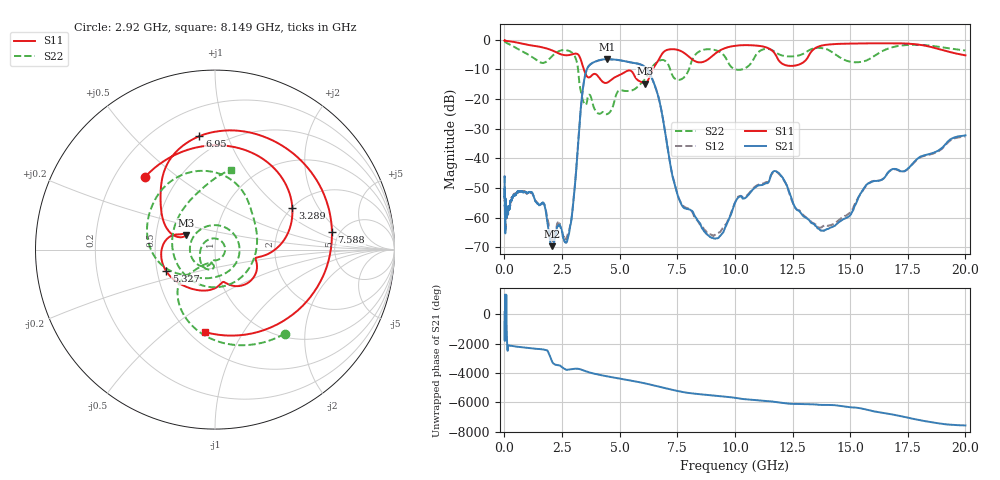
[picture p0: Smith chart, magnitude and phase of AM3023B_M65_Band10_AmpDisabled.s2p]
!Agilent Technologies,E8364B,MY43040894,A.07.50.67
!Agilent E8364B: A.07.50.67
!Date: Tuesday, October 27, 2020 10:50:51
!Correction: S11(Full 2 Port(1,2))
!S21(Full 2 Port(1,2))
!S12(Full 2 Port(1,2))
!S22(Full 2 Port(1,2))
!S2P File: Measurements: S11, S21, S12, S22:Log Frequency Sweep
# Hz S  dB  R 50
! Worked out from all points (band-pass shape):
!   3201 points, 10 MHz to 20 GHz, reference 50 ohm
!   highest |S21| = -6.60 dB at 4.447 GHz (marker M1); lowest = -69.6 dB at 2.06 GHz (marker M2)
!   |S21| within 3 dB of the highest: 3.602 GHz to 6.153 GHz (2.55 GHz wide, 52.3 % of centre)
!   lowest |S11| = -14.8 dB at 6.099 GHz (marker M3), VSWR 1.44, Z = 35.6 + j5.94 ohm
!   |S11| at or under -10 dB: 3.445 GHz to 6.435 GHz (2.99 GHz wide, 60.5 % of centre)
!   |S22| runs from -25.2 to -0.6 dB; largest |S21 - S12| = 0.0089
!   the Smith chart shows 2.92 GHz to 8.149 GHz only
!   S11 on the Smith chart (normalised r, x): 2.92 GHz: 0.33, +0.38; 3.289 GHz: 2.02, +1.22; 5.327 GHz: 0.56, -0.15; 6.95 GHz: 0.38, +0.80; 7.588 GHz: 4.33, +1.48; 8.149 GHz: 0.59, -0.70
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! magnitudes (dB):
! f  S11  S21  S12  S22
! 10 MHz  -0.3  -46.2  -45.8  -0.6
! 35.55 MHz  -0.3  -63.9  -63.7  -0.7
! 48.3 MHz  -0.3  -53.5  -57.0  -0.9
! 126.1 MHz  -0.5  -58.4  -58.4  -1.3
! 447.2 MHz  -0.8  -52.4  -52.2  -2.5
! 1.59 GHz  -2.5  -55.5  -55.4  -7.8
! 2.06 GHz  -3.6  -69.6  -67.6  -5.7
! 2.694 GHz  -5.3  -68.4  -66.7  -3.6
! 2.92 GHz  -5.0  -59.7  -60.0  -4.3
! 3.289 GHz  -6.2  -25.6  -25.6  -16.3
! 3.608 GHz  -12.6  -9.5  -9.6  -19.6
! 4.447 GHz  -14.5  -6.6  -6.6  -25.1
! 5.327 GHz  -10.5  -7.5  -7.5  -17.3
! 5.639 GHz  -12.1  -7.9  -7.9  -16.8
! 6.099 GHz  -14.8  -9.2  -9.2  -13.3
! 6.95 GHz  -3.9  -30.0  -29.9  -7.0
! 7.588 GHz  -3.6  -54.0  -53.8  -13.5
! 8.149 GHz  -6.7  -57.8  -58.1  -6.8
! 9.198 GHz  -4.4  -67.0  -65.4  -3.7
! 11.78 GHz  -5.2  -44.4  -44.5  -4.3
! 14.11 GHz  -1.6  -63.6  -62.6  -3.7
! 20 GHz  -5.3  -32.3  -32.6  -3.7
